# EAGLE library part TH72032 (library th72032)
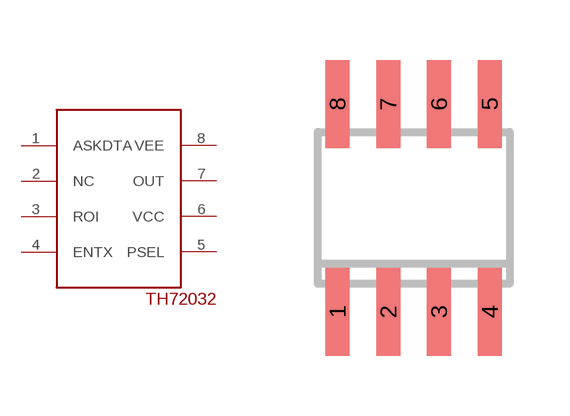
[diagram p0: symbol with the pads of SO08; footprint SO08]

Designator prefix -

## TH72032NORMAL  [SO08]
1  ASKDTA
2  NC
3  ROI
4  ENTX
5  PSEL
6  VCC
7  OUT
8  VEE

## Footprint SO08 (pad centres in mm)
Small Outline Package 8 NS Package M08A
smd 0.6 x 2.2: 1 -1.905,-2.6; 2 -0.635,-2.6; 3 0.635,-2.6; 4 1.905,-2.6; 5 1.905,2.6; 6 0.635,2.6; 7 -0.635,2.6; 8 -1.905,2.6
